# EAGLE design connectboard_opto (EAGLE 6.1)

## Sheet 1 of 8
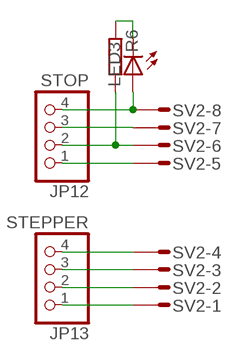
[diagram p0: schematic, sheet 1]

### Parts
JP12  STOP  PINHD-1X04_2.54-S  [1X04-S]
JP13  STEPPER  PINHD-1X04_2.54-S  [1X04-S]
LED3  LED3MM  [LED3MM]
R6  R-EU0207/10  [0207/10]
SV2  ML10E  [ML10]

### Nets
MYZ-1: JP13.1 SV2.1
MYZ-2: JP13.2 SV2.2
MYZ-3: JP13.3 SV2.3
MYZ-4: JP13.4 SV2.4
N$5: LED3.K(C) R6.1
YZ-LEDA: JP12.4 LED3.A SV2.8
YZ-LEDC: JP12.3 SV2.7
YZ-SW: JP12.2 R6.2 SV2.6
YZ-SW-GND: JP12.1 SV2.5
Unconnected: SV2.9 SV2.10

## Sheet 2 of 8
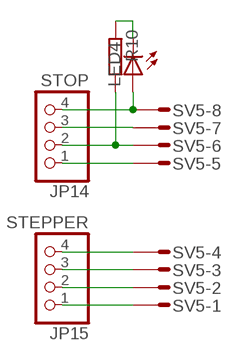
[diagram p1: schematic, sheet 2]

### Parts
JP14  STOP  PINHD-1X04_2.54-S  [1X04-S]
JP15  STEPPER  PINHD-1X04_2.54-S  [1X04-S]
LED4  LED3MM  [LED3MM]
R10  R-EU0207/10  [0207/10]
SV5  ML10E  [ML10]

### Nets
MYZ-5: JP15.1 SV5.1
MYZ-6: JP15.2 SV5.2
MYZ-7: JP15.3 SV5.3
MYZ-8: JP15.4 SV5.4
N$6: LED4.K(C) R10.1
YZ-LEDA1: JP14.4 LED4.A SV5.8
YZ-LEDC1: JP14.3 SV5.7
YZ-SW1: JP14.2 R10.2 SV5.6
YZ-SW-GND1: JP14.1 SV5.5
Unconnected: SV5.9 SV5.10

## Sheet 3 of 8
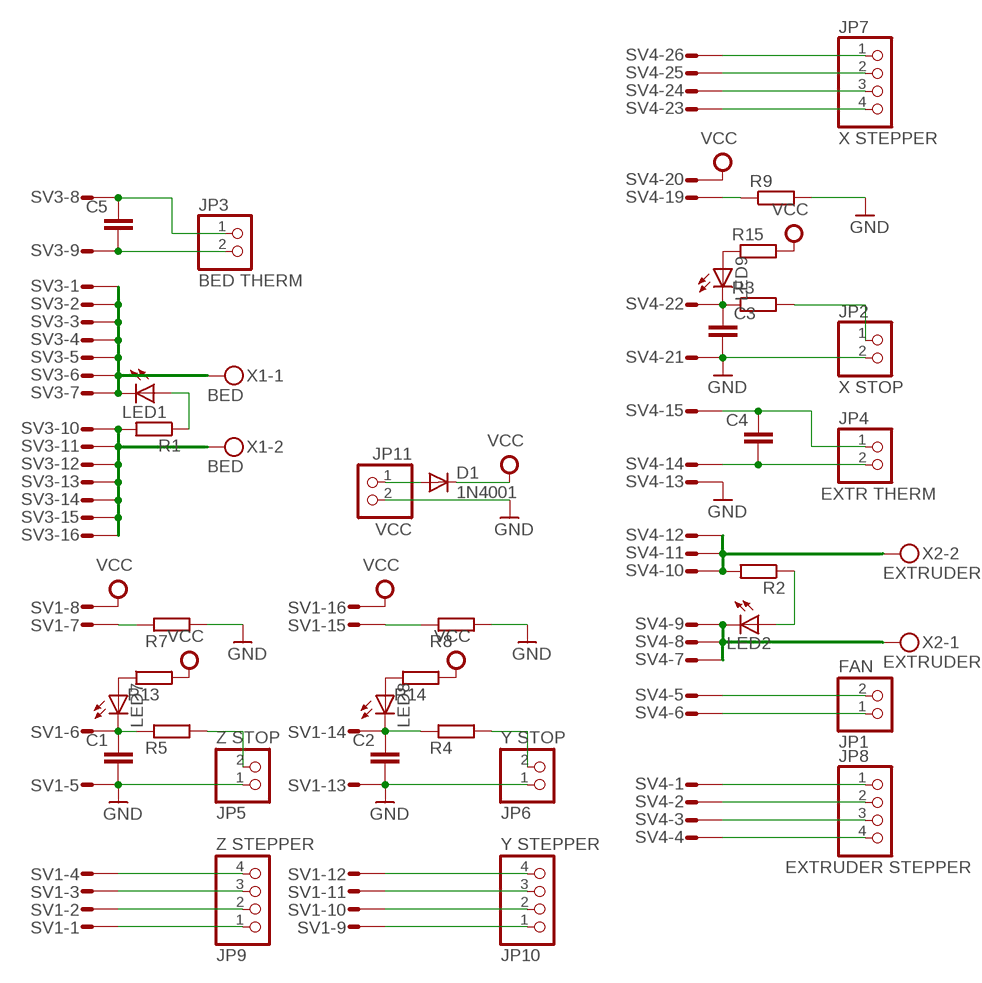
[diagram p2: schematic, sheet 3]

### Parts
C1  C-EU025-024X044  [C025-024X044]
C2  C-EU025-024X044  [C025-024X044]
C3  C-EU025-024X044  [C025-024X044]
C4  C-EU025-024X044  [C025-024X044]
C5  C-EU025-024X044  [C025-024X044]
D1  1N4001  [DO41-10]
JP1  FAN  PINHD-1X02_2.54-S  [1X02-S]
JP2  X STOP  PINHD-1X02_2.54  [1X02]
JP3  BED THERM  PINHD-1X02_2.54  [1X02]
JP4  EXTR THERM  PINHD-1X02_2.54  [1X02]
JP5  Z STOP  PINHD-1X02_2.54-S  [1X02-S]
JP6  Y STOP  PINHD-1X02_2.54-S  [1X02-S]
JP7  X STEPPER  PINHD-1X04_2.54-S  [1X04-S]
JP8  EXTRUDER STEPPER  PINHD-1X04_2.54-S  [1X04-S]
JP9  Z STEPPER  PINHD-1X04_2.54-S  [1X04-S]
JP10  Y STEPPER  PINHD-1X04_2.54-S  [1X04-S]
JP11  VCC  PINHD-1X02_2.54-S  [1X02-S]
LED1  LED3MM  [LED3MM]
LED2  LED3MM  [LED3MM]
LED7  LED3MM  [LED3MM]
LED8  LED3MM  [LED3MM]
LED9  LED3MM  [LED3MM]
R1  R-EU0207/10  [0207/10]
R2  R-EU0207/10  [0207/10]
R3  R-EU0207/2V  [0207/2V]
R4  R-EU0207/2V  [0207/2V]
R5  R-EU0207/2V  [0207/2V]
R7  R-EU0207/2V  [0207/2V]
R8  R-EU0207/2V  [0207/2V]
R9  R-EU0207/2V  [0207/2V]
R13  R-EU0207/2V  [0207/2V]
R14  R-EU0207/2V  [0207/2V]
R15  R-EU0207/10  [0207/10]
SV1  ML16E  [ML16]
SV3  ML16E  [ML16]
SV4  ML26E  [ML26]
X1  BED  MKDSN1,5/2-5,08  [MKDSN1,5/2-5,08]
X2  EXTRUDER  MKDSN1,5/2-5,08  [MKDSN1,5/2-5,08]

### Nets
GND: C1.2 C2.2 C3.2 JP2.2 JP5.1 JP6.1 JP11.2 R7.2 R8.2 R9.2 SV1.5 SV1.13 SV4.13 SV4.21
MEXT-1: JP8.1 SV4.1
MEXT-2: JP8.2 SV4.2
MEXT-3: JP8.3 SV4.3
MEXT-4: JP8.4 SV4.4
MX-1: JP7.1 SV4.26
MX-2: JP7.2 SV4.25
MX-3: JP7.3 SV4.24
MX-4: JP7.4 SV4.23
MY-1: JP10.1 SV1.9
MY-2: JP10.2 SV1.10
MY-3: JP10.3 SV1.11
MY-4: JP10.4 SV1.12
MZ-1: JP9.1 SV1.1
MZ-2: JP9.2 SV1.2
MZ-3: JP9.3 SV1.3
MZ-4: JP9.4 SV1.4
N$1: C5.2 JP3.2 SV3.9
N$2: C5.1 JP3.1 SV3.8
N$3: LED1.K(C) SV3.1 SV3.2 SV3.3 SV3.4 SV3.5 SV3.6 SV3.7 X1.1
N$4: R1.2 SV3.10 SV3.11 SV3.12 SV3.13 SV3.14 SV3.15 SV3.16 X1.2
N$9: JP5.2 R5.2
N$11: JP6.2 R4.2
N$21: C4.2 JP4.2 SV4.14
N$22: C4.1 JP4.1 SV4.15
N$23: JP1.1 SV4.6
N$24: JP1.2 SV4.5
N$25: R2.2 SV4.10 SV4.11 SV4.12 X2.2
N$26: LED7.A R13.1
N$27: LED8.A R14.1
N$28: D1.A JP11.1
N$29: LED9.A R15.1
N$30: JP2.1 R3.2
N$32: LED2.K(C) SV4.7 SV4.8 SV4.9 X2.1
N$33: LED1.A R1.1
N$34: LED2.A R2.1
VCC: D1.C R13.2 R14.2 R15.2 SV1.8 SV1.16 SV4.20
X-LEDC: R9.1 SV4.19
X-SW: C3.1 LED9.K(C) R3.1 SV4.22
Y-LEDC: R8.1 SV1.15
Y-SW: C2.1 LED8.K(C) R4.1 SV1.14
Z-LEDC: R7.1 SV1.7
Z-SW: C1.1 LED7.K(C) R5.1 SV1.6
Unconnected: SV4.16 SV4.17 SV4.18

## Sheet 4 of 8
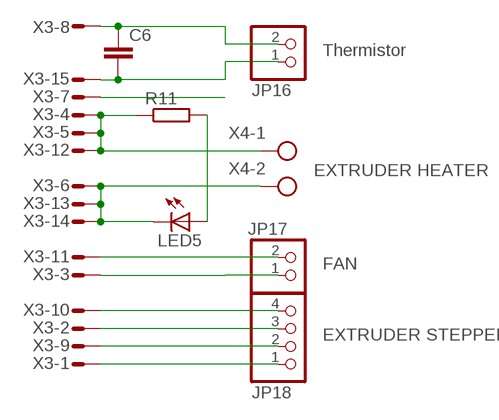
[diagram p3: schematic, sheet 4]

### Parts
C6  C-EU025-024X044  [C025-024X044]
JP16  Thermistor  PINHD-1X02_2.54-90°-S  [1X02/90-S]
JP17  FAN  PINHD-1X02_2.54-90°-S  [1X02/90-S]
JP18  EXTRUDER STEPPER  PINHD-1X04_2.54-90°-S  [1X04/90-S]
LED5  LED3MM  [LED3MM]
R11  R-EU0207/10  [0207/10]
X3  M15HS  [M15H]
X4  EXTRUDER HEATER  MKDSN1,5/2-5,08  [MKDSN1,5/2-5,08]

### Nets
N$7: JP18.1 X3.1
N$8: JP18.3 X3.2
N$10: JP18.2 X3.9
N$12: JP18.4 X3.10
N$13: JP17.1 X3.3
N$14: JP17.2 X3.11
N$15: C6.2 JP16.1 X3.15
N$16: C6.1 JP16.2 X3.8
N$17: R11.1 X3.4 X3.5 X3.12 X4.1
N$18: LED5.K(C) X3.6 X3.13 X3.14 X4.2
N$19: LED5.A R11.2
SHIELD: X3.7

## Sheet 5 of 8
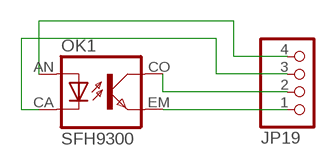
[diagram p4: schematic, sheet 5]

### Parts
JP19  PINHD-1X04_2.54-90°L-S  [1X04/90L-S]
OK1  SFH9300  [SFH9300]

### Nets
LEDA: JP19.4 OK1.AN(A)
LEDC: JP19.3 OK1.CA(C)
SW: JP19.2 OK1.CO(COL)
SW-GND: JP19.1 OK1.EM(EMIT)

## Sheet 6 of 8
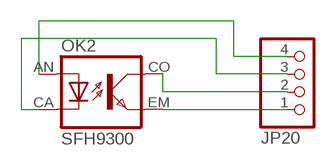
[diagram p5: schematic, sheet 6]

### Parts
JP20  PINHD-1X04_2.54-90°L-S  [1X04/90L-S]
OK2  SFH9300  [SFH9300]

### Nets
LEDA1: JP20.4 OK2.AN(A)
LEDC1: JP20.3 OK2.CA(C)
SW1: JP20.2 OK2.CO(COL)
SW-GND1: JP20.1 OK2.EM(EMIT)

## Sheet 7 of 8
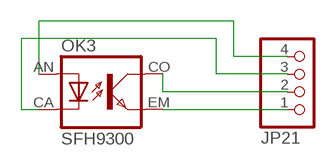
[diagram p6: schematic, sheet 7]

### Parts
JP21  PINHD-1X04_2.54-90°L-S  [1X04/90L-S]
OK3  SFH9300  [SFH9300]

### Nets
LEDA2: JP21.4 OK3.AN(A)
LEDC2: JP21.3 OK3.CA(C)
SW2: JP21.2 OK3.CO(COL)
SW-GND2: JP21.1 OK3.EM(EMIT)

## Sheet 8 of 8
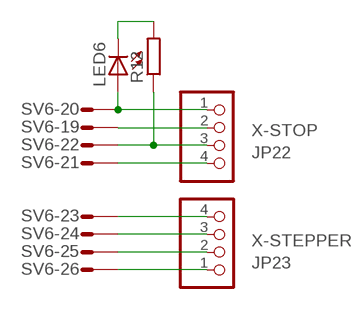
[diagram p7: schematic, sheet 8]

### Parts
JP22  X-STOP  PINHD-1X04_2.54-90°L-S  [1X04/90L-S]
JP23  X-STEPPER  PINHD-1X04_2.54-90°-S  [1X04/90-S]
LED6  LED3MM  [LED3MM]
R12  R-EU0207/10  [0207/10]
SV6  ML26LE  [ML26L]

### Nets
N$20: LED6.K(C) R12.2
X-LEDA: JP22.1 LED6.A SV6.20
X-LEDC1: JP22.2 SV6.19
X-SW1: JP22.3 R12.1 SV6.22
X-SW-GND: JP22.4 SV6.21
XM1: JP23.1 SV6.26
XM2: JP23.2 SV6.25
XM3: JP23.3 SV6.24
XM4: JP23.4 SV6.23
Unconnected: SV6.1 SV6.2 SV6.3 SV6.4 SV6.5 SV6.6 SV6.7 SV6.8 SV6.9 SV6.10 SV6.11 SV6.12 SV6.13 SV6.14 SV6.15 SV6.16 SV6.17 SV6.18

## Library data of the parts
C1-C6 = rcl-2:C-EU: CAPACITOR, European symbol
D1 = diode:1N400*: DIODE
JP1-JP6 JP11 JP16 JP17 = con-pinhead-2:PINHD-1X02: PIN HEADER
JP7-JP10 JP12-JP15 JP18-JP23 = con-pinhead-2:PINHD-1X04: PIN HEADER
LED1-LED9 = led:LED: LED
OK1-OK3 = opto-siemens:SFH9*: Slotted Interrupter / Gabellichtschranke Source: http://www.osram.convergy.de/
R1-R15 = rcl-2:R-EU: RESISTOR, European symbol
SV1 SV3 = con-dil:ML16?E: HARTING
SV2 SV5 = con-dil:ML10?E: HARTING
SV4 SV6 = con-dil:ML26?E: HARTING
X1 X2 X4 = con-phoenix-508:MKDSN1,5/2-5,08: MKDSN 1,5/ 2-5,08 Printklemme
X3 = con-subd:M15?S: SUB-D

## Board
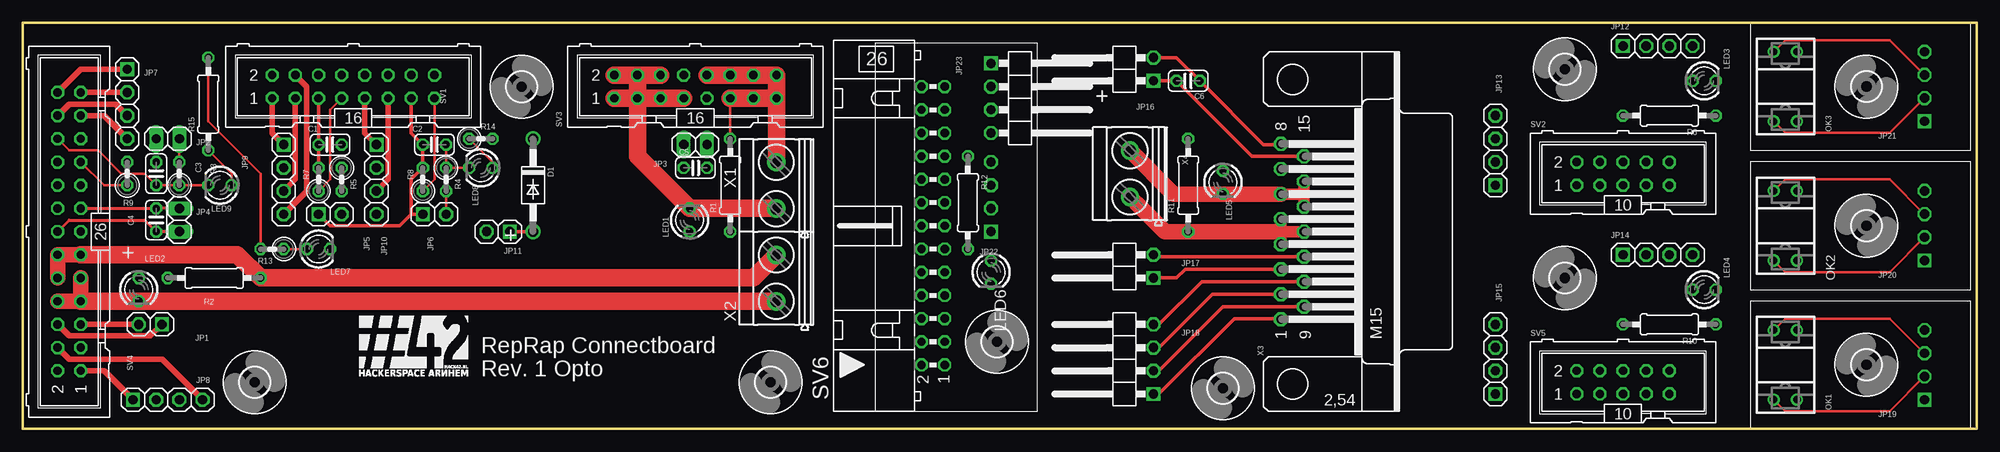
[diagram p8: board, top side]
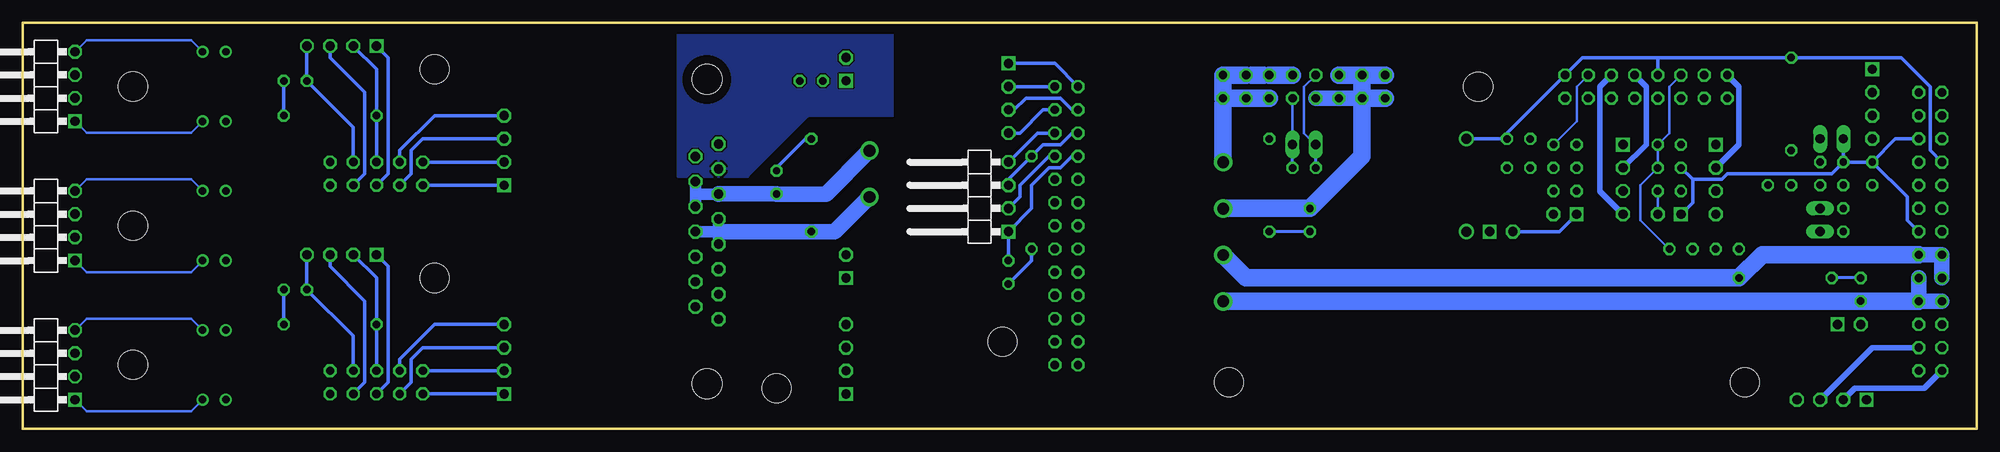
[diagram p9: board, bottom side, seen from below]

Size 214 x 44.45 mm. Coordinates in mm from the lower left corner, seen from the top.
Outline: 0,0 214,0 214,44.45 0,44.45 0,0
Copper layers (1*16): Top 0.035mm / dielectric 1.5mm / Bottom 0.035mm
Design rules: minimum track width 10mil, minimum drill 24mil, track to track 8mil, track to pad 8mil, pad to pad 8mil, via to via 8mil, smd to smd 8mil, copper to edge 40mil, drill to drill 8mil, minimum pad ring 10mil, minimum via ring 8mil, stop-mask expansion 4mil, vias tented up to drill 0mil, thermal gap 10mil

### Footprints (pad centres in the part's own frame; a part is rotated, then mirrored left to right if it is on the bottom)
C025-024X044 = drill 0.813 octagon: 1 -1.27,0; 2 1.27,0
DO41-10 = drill 1.118: A 5.08,0; C -5.08,0
1X02-S = drill 1.016 square: 1 -1.27,0 | drill 1.016 octagon: 2 1.27,0
1X02 = drill 1.016 long: 1 -1.27,0; 2 1.27,0
1X04-S = drill 1.016 square: 1 -3.81,0 | drill 1.016 octagon: 2 -1.27,0; 3 1.27,0; 4 3.81,0
1X02/90-S = drill 1.016 square: 1 -2.54,-3.81 | drill 1.016 octagon: 2 0,-3.81
1X04/90-S = drill 1.016 square: 1 -3.81,-3.81 | drill 1.016 octagon: 2 -1.27,-3.81; 3 1.27,-3.81; 4 3.81,-3.81
1X04/90L-S = drill 1.016 square: 1 3.81,-3.81 | drill 1.016 octagon: 2 1.27,-3.81; 3 -1.27,-3.81; 4 -3.81,-3.81
LED3MM = drill 0.813 octagon: A -1.27,0; K 1.27,0
SFH9300 = drill 0.813: AN -3.81,1.27; CA -3.81,-1.27; CO 3.81,-1.27; EM 3.81,1.27
0207/10 = drill 0.813 octagon: 1 -5.08,0; 2 5.08,0
0207/2V = drill 0.813 octagon: 1 -1.27,0; 2 1.27,0
ML16 = drill 0.914 octagon: 1 -8.89,-1.27; 2 -8.89,1.27; 3 -6.35,-1.27; 4 -6.35,1.27; 5 -3.81,-1.27; 6 -3.81,1.27; 7 -1.27,-1.27; 8 -1.27,1.27; 9 1.27,-1.27; 10 1.27,1.27; 11 3.81,-1.27; 12 3.81,1.27; 13 6.35,-1.27; 14 6.35,1.27; 15 8.89,-1.27; 16 8.89,1.27
ML10 = drill 0.914 octagon: 1 -5.08,-1.27; 2 -5.08,1.27; 3 -2.54,-1.27; 4 -2.54,1.27; 5 0,-1.27; 6 0,1.27; 7 2.54,-1.27; 8 2.54,1.27; 9 5.08,-1.27; 10 5.08,1.27
ML26 = drill 0.914 octagon: 1 -15.24,-1.27; 2 -15.24,1.27; 3 -12.7,-1.27; 4 -12.7,1.27; 5 -10.16,-1.27; 6 -10.16,1.27; 7 -7.62,-1.27; 8 -7.62,1.27; 9 -5.08,-1.27; 10 -5.08,1.27; 11 -2.54,-1.27; 12 -2.54,1.27; 13 0,-1.27; 14 0,1.27; 15 2.54,-1.27; 16 2.54,1.27; 17 5.08,-1.27; 18 5.08,1.27; 19 7.62,-1.27; 20 7.62,1.27; 21 10.16,-1.27; 22 10.16,1.27; 23 12.7,-1.27; 24 12.7,1.27; 25 15.24,-1.27; 26 15.24,1.27
ML26L = drill 0.914 octagon: 1 -15.24,-1.27; 2 -15.24,1.27; 3 -12.7,-1.27; 4 -12.7,1.27; 5 -10.16,-1.27; 6 -10.16,1.27; 7 -7.62,-1.27; 8 -7.62,1.27; 9 -5.08,-1.27; 10 -5.08,1.27; 11 -2.54,-1.27; 12 -2.54,1.27; 13 0,-1.27; 14 0,1.27; 15 2.54,-1.27; 16 2.54,1.27; 17 5.08,-1.27; 18 5.08,1.27; 19 7.62,-1.27; 20 7.62,1.27; 21 10.16,-1.27; 22 10.16,1.27; 23 12.7,-1.27; 24 12.7,1.27; 25 15.24,-1.27; 26 15.24,1.27
3,2 = hole 3.2: 0,0
MKDSN1,5/2-5,08 = drill 1.3 pad 2: 1 -2.561,0.025; 2 2.519,0.025
M15H = drill 1.016 octagon: 1 -9.601,1.27; 2 -6.858,1.27; 3 -4.115,1.27; 4 -1.372,1.27; 5 1.372,1.27; 6 4.115,1.27; 7 6.858,1.27; 8 9.601,1.27; 9 -8.23,-1.27; 10 -5.486,-1.27; 11 -2.743,-1.27; 12 0,-1.27; 13 2.743,-1.27; 14 5.486,-1.27; 15 8.23,-1.27 | hole 3.302: 16.662,0; -16.662,0

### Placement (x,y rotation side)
C1  33.66,31.11 180 top
C2  45.09,31.11 180 top
C3  14.61,27.94 90 top
C4  14.61,22.86 270 top
C5  73.66,28.57 0 top
C6  127.64,38.1 180 top
D1  55.88,26.67 270 top
JP1  13.97,11.43 180 top
JP2  15.88,31.75 180 top
JP3  73.66,31.11 0 top
JP4  17.14,22.86 270 top
JP5  33.66,23.5 0 top
JP6  45.09,23.5 0 top
JP7  11.43,35.56 270 top
JP8  15.88,3.17 0 top
JP9  28.57,27.3 270 top
JP10  38.73,27.3 270 top
JP11  52.07,21.59 180 top
JP12  179.07,41.91 0 top
JP13  161.29,30.48 90 top
JP14  179.07,19.05 0 top
JP15  161.29,7.62 90 top
JP16  120.02,40.64 90 top
JP17  120.02,19.05 90 top
JP18  120.02,7.62 90 top
JP19  212.09,7 270 top
JP20  212.09,22.23 270 top
JP21  212.09,37.48 270 top
JP22  109.86,25.4 270 top
JP23  109.86,36.2 270 top
LED1  73.03,22.86 90 top
LED2  12.7,15.24 270 top
LED3  184.15,38.1 0 top
LED4  184.15,15.24 0 top
LED5  131.44,26.99 270 top
LED6  106.05,17.14 270 top
LED7  32.38,19.68 0 top
LED8  50.16,28.57 180 top
LED9  21.59,26.67 180 top
OK1  193.04,7 270 top
OK2  193.04,22.23 270 top
OK3  193.04,37.48 270 top
R1  77.47,26.67 90 top
R2  20.95,16.51 0 top
R3  17.14,27.94 90 top
R4  46.35,27.3 270 top
R5  34.92,27.3 270 top
R6  180.34,34.29 180 top
R7  32.38,27.3 90 top
R8  43.81,27.3 90 top
R9  11.43,27.94 90 top
R10  180.34,11.43 180 top
R11  127.64,26.67 90 top
R12  103.5,24.77 270 top
R13  27.3,19.68 180 top
R14  50.16,31.75 0 top
R15  20.32,35.56 90 top
SV1  36.2,37.47 0 top
SV2  175.26,27.94 0 top
SV3  73.66,37.47 0 top
SV4  5.08,21.59 90 top
SV5  175.26,5.08 0 top
SV6  99.69,22.23 90 top
U$1  [3,2]  25.4,5.08 0 top
U$2  [3,2]  81.92,5.08 0 top
U$3  [3,2]  168.91,39.37 90 top
U$4  [3,2]  54.61,37.47 0 top
U$5  [3,2]  168.91,16.51 90 top
U$6  [3,2]  131.44,4.45 0 top
U$7  [3,2]  201.93,7 90 top
U$8  [3,2]  201.93,22.23 90 top
U$9  [3,2]  201.93,37.48 90 top
U$10  [3,2]  106.68,9.53 0 top
U$11  [LOGO_HACK42-12X7]  36.83,5.71 0 top
X1  82.55,26.67 90 top
X2  82.55,16.51 90 top
X3  139.06,21.59 90 top
X4  121.28,27.94 90 top

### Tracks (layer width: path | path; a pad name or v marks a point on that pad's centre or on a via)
GND
  Top 0.406: SV1.13 42.55,32.38 C2.2 R8.2 42.55,27.3 42.55,23.5 | R7.2 C1.2 SV1.5 | JP5.1 33.66,22.23 41.27,22.23 42.55,23.5 | JP6.1 42.55,23.5
  Bottom 0.406: C3.2 R9.2 | SV4.21 8.89,31.75 R9.2 | C3.2 JP2.2 | 31.11,27.3 R7.2 | 31.11,27.3 31.11,24.77 JP5.1 | C3.2 15.88,27.94 27.3,27.94 27.94,27.3 31.11,27.3 | JP11.2 45.72,21.59 JP6.1 | R9.2 7.62,25.4 7.62,22.86 SV4.13
LEDA
  Bottom 0.254: OK1.AN 195.58,12.07 207.01,12.07 JP19.4
LEDA1
  Bottom 0.254: OK2.AN 195.58,27.32 207.01,27.32 JP20.4
LEDA2
  Bottom 0.254: OK3.AN 195.58,42.55 207.01,42.55 JP21.4
LEDC
  Top 0.254: OK1.CA 193.04,12.07 204.47,12.07 JP19.3
LEDC1
  Top 0.254: OK2.CA 193.04,27.32 204.47,27.32 JP20.3
LEDC2
  Top 0.254: OK3.CA 193.04,42.55 204.47,42.55 JP21.3
MEXT-1
  Top 0.61: SV4.1 8.89,6.35 JP8.1
MEXT-2
  Bottom 0.61: SV4.2 5.71,4.45 13.34,4.45 JP8.2
MEXT-3
  Bottom 0.61: SV4.3 11.43,8.89 JP8.3
MEXT-4
  Top 0.61: SV4.4 5.08,7.62 15.24,7.62 JP8.4
MX-1
  Top 0.61: SV4.26 6.35,39.37 JP7.1
MX-2
  Top 0.61: JP7.2 SV4.25
MX-3
  Top 0.61: SV4.24 5.08,35.56 10.16,35.56 JP7.3
MX-4
  Top 0.61: SV4.23 8.89,34.29 JP7.4
MY-1
  Top 0.61: SV1.9 37.47,32.38 JP10.1
MY-2
  Bottom 0.61: SV1.10 36.2,37.47 36.2,31.11 JP10.2
MY-3
  Top 0.61: SV1.11 40.01,27.3 JP10.3
MY-4
  Bottom 0.61: SV1.12 41.27,37.47 41.27,26.04 JP10.4
MYZ-1
  Bottom 0.406: SV2.1 JP13.1
MYZ-2
  Bottom 0.406: JP13.2 SV2.2
MYZ-3
  Bottom 0.406: JP13.3 170.18,31.75 171.45,30.48 171.45,27.94 SV2.3
MYZ-4
  Bottom 0.406: JP13.4 168.91,34.29 172.72,30.48 SV2.4
MYZ-5
  Bottom 0.406: SV5.1 JP15.1
MYZ-6
  Bottom 0.406: JP15.2 SV5.2
MYZ-7
  Bottom 0.406: JP15.3 170.18,8.89 171.45,7.62 171.45,5.08 SV5.3
MYZ-8
  Bottom 0.406: JP15.4 168.91,11.43 172.72,7.62 SV5.4
MZ-1
  Top 0.61: SV1.1 27.3,32.38 JP9.1
MZ-2
  Bottom 0.61: SV1.2 26.04,37.47 26.04,31.11 JP9.2
MZ-3
  Top 0.61: SV1.3 29.84,27.3 JP9.3
MZ-4
  Top 0.61: SV1.4 31.11,37.47 31.11,26.04 JP9.4
N$1
  Bottom 0.254: JP3.2 SV3.9
  Bottom 0.305: C5.2 JP3.2
N$2
  Bottom 0.254: SV3.8 73.66,37.47 73.66,32.38 JP3.1
  Bottom 0.305: C5.1 JP3.1
N$3
  Top 1.93: SV3.2 SV3.4 | SV3.4 SV3.6 | SV3.1 SV3.3 | SV3.3 SV3.7 | SV3.4 SV3.3 | SV3.3 67.31,29.84 LED1.K 82.55,24.13
  Bottom 1.27: 66.67,36.2 SV3.3 SV3.5 SV3.7 | 82.55,24.13 X1.1
  Bottom 1.676: SV3.7 SV3.3
  Bottom 1.93: SV3.4 SV3.6 | SV3.1 SV3.3 | SV3.4 SV3.3 | SV3.4 SV3.2 | SV3.3 67.31,29.84 LED1.K 82.55,24.13
N$4
  Top 0.254: SV3.11 R1.2
  Top 1.93: 82.55,29.21 SV3.15 | SV3.15 SV3.16 SV3.14 SV3.12 SV3.10 | SV3.11 SV3.13 SV3.15
  Bottom 0.406: 82.55,29.21 82.53,29.21 X1.2
  Bottom 1.27: 79.38,38.73 SV3.14 | SV3.12 78.11,38.73 | 82.55,35.56 SV3.15 | 82.55,29.21 X1.2
  Bottom 1.93: SV3.11 SV3.13 SV3.15 SV3.16 SV3.14 | SV3.10 SV3.12 | 78.11,38.73 79.38,38.73 | 82.55,29.21 82.55,35.56
N$5
  Bottom 0.406: R6.1 LED3.K
N$6
  Bottom 0.406: R10.1 LED4.K
N$7
  Top 0.406: JP18.1 124.46,3.81 132.72,12.06 137.79,12.06 X3.1
N$8
  Top 0.406: JP18.3 124.46,8.89 130.3,14.73 X3.2 137.92,14.73
N$9
  Bottom 0.254: JP5.2 R5.2
N$10
  Top 0.254: 140.34,13.34 X3.9
  Top 0.406: JP18.2 124.46,6.35 131.44,13.34 140.34,13.34
N$11
  Top 0.254: JP6.2 R4.2
N$12
  Top 0.406: JP18.4 124.46,11.43 129.13,16.1 X3.10
N$13
  Top 0.406: X3.3 127.33,17.48 126.36,16.51 JP17.1
N$14
  Top 0.406: JP17.2 124.26,18.85 X3.11
N$15
  Top 0.254: 140.34,29.84 X3.15
  Top 0.406: JP16.1 C6.2 134.62,29.84 140.34,29.84
N$16
  Top 0.254: 137.79,31.11 X3.8
  Top 0.406: JP16.2 126.36,40.64 C6.1 135.89,31.11 137.79,31.11
N$17
  Top 0.254: 137.79,20.32 X3.4
  Top 0.813: 137.79,22.86 X3.5
  Top 1.27: 137.79,21.59 137.79,20.32 | 137.79,21.59 X3.12 | 137.79,21.59 137.79,22.86
  Top 1.676: X4.1 121.92,24.77 125.09,21.59 R11.1 137.79,21.59
  Bottom 1.27: 137.79,21.59 137.79,22.86 | 137.79,21.59 137.79,20.32 | X3.12 137.79,21.59
  Bottom 1.676: 121.28,25.4 125.09,21.59 137.79,21.59
N$18
  Top 0.254: LED5.K 131.44,25.7
  Top 0.813: 121.28,30.48 X4.2
  Top 1.27: X3.14 140.34,25.7 | X3.13 140.34,25.7 | 140.34,25.7 X3.6
  Top 1.676: 121.28,30.48 126.03,25.7 131.44,25.7 X3.6
  Bottom 0.254: 130.18,25.08 130.18,25.7 | 121.44,30.32 121.28,30.16 X4.2
  Bottom 1.27: 140.34,24.13 140.34,25.7 | X3.6 140.34,25.7 | 140.34,25.7 X3.14
  Bottom 1.676: LED5.K 137.78,25.72 X3.6 | 131.44,25.7 130.18,25.7 126.03,25.7 121.44,30.32 121.28,30.48
N$19
  Bottom 0.406: R11.2 128.27,31.75 131.44,28.57 LED5.A
N$20
  Bottom 0.406: R12.2 103.5,18.41 LED6.K
N$21
  Top 0.305: JP4.2 C4.2 13.34,22.86 5.08,22.86 SV4.14
N$22
  Top 0.305: JP4.1 C4.1 SV4.15
N$23
  Top 0.61: SV4.6 5.08,10.16 13.97,10.16 JP1.1
N$24
  Top 0.61: JP1.2 SV4.5
N$25
  Top 1.676: SV4.10 SV4.12 SV4.11
  Top 1.93: 82.55,19.05 80.01,16.51 R2.2 23.5,19.05 SV4.11
  Bottom 1.676: SV4.11 SV4.12 SV4.10
  Bottom 1.93: SV4.11 23.5,19.05 R2.2 80.01,16.51 81.92,18.41 X2.2
N$26
  Top 0.254: R13.1 LED7.A
N$27
  Top 0.254: R14.1 51.44,29.21 LED8.A
N$28
  Top 0.406: D1.A JP11.1
N$29
  Top 0.254: LED9.A 22.86,27.94 R15.1
N$30
  Top 0.254: JP2.1 R3.2
N$32
  Top 1.676: SV4.9 SV4.7 SV4.8
  Top 1.93: SV4.7 LED2.K 82.55,13.97
  Bottom 1.676: SV4.9 SV4.7 SV4.8
  Bottom 1.93: SV4.7 LED2.K 81.92,13.97 X2.1
N$33
  Bottom 0.305: LED1.A R1.1
N$34
  Bottom 0.305: LED2.A R2.1
SHIELD
  pour Bottom: 118.75,34.29 127.95,34.29 134.62,27.62 142.24,27.62 142.24,43.18 118.75,43.18
SW
  Top 0.254: OK1.CO 193.04,1.92 204.47,1.92 JP19.2
SW1
  Top 0.254: OK2.CO 193.04,17.16 204.47,17.16 JP20.2
SW2
  Top 0.254: OK3.CO 193.04,32.4 204.47,32.4 JP21.2
SW-GND
  Bottom 0.254: OK1.EM 195.58,1.92 207.01,1.92 JP19.1
SW-GND1
  Bottom 0.254: OK2.EM 195.58,17.16 207.01,17.16 JP20.1
SW-GND2
  Bottom 0.254: OK3.EM 195.58,32.4 207.01,32.4 JP21.1
VCC
  Top 0.254: R13.2 26.04,27.94 20.32,33.66 R15.2
  Bottom 0.406: SV4.20 5.08,30.48 5.08,37.47 8.26,40.64 R15.2 34.92,40.64 | SV1.8 34.92,40.64 | 34.92,40.64 43.18,40.64 SV1.16 51.44,32.38 R14.2 D1.C
X-LEDA
  Bottom 0.406: SV6.20 99.06,29.84 100.33,28.57 101.6,28.57 103.5,26.67 103.5,24.13 JP22.1 LED6.A
X-LEDC
  Top 0.254: R9.1 8.89,26.67 SV4.19
X-LEDC1
  Bottom 0.406: JP22.2 104.78,25.4 104.78,26.67 101.6,29.84 SV6.19
X-SW
  Top 0.254: SV4.22 5.08,30.48 8.26,30.48 10.79,27.94 13.34,27.94 C3.1 R3.1 LED9.K
X-SW1
  Bottom 0.406: JP22.3 106.05,27.3 R12.1 102.23,31.11 100.33,31.11 99.06,32.38 SV6.22
X-SW-GND
  Bottom 0.406: JP22.4 102.87,32.38 SV6.21
XM1
  Bottom 0.406: SV6.26 100.97,40.01 JP23.1
XM2
  Bottom 0.406: JP23.2 SV6.25
XM3
  Bottom 0.406: JP23.3 105.41,34.92 104.14,36.2 100.33,36.2 99.06,34.92 SV6.24
XM4
  Bottom 0.406: SV6.23 102.23,34.92 104.78,32.38 JP23.4
Y-LEDC
  Top 0.254: R8.1 45.09,27.3 SV1.15
Y-SW
  Top 0.254: C2.1 R4.1 LED8.K
  Bottom 0.254: SV1.14 43.81,37.47 43.81,33.66 C2.1
YZ-LEDA
  Bottom 0.406: JP12.4 LED3.A 177.8,33.02 SV2.8
YZ-LEDA1
  Bottom 0.406: JP14.4 LED4.A 177.8,10.16 SV5.8
YZ-LEDC
  Bottom 0.406: JP12.3 180.34,40.64 176.53,36.83 176.53,27.94 SV2.7
YZ-LEDC1
  Bottom 0.406: JP14.3 180.34,17.78 176.53,13.97 176.53,5.08 SV5.7
YZ-SW
  Bottom 0.406: JP12.2 175.26,39.37 R6.2 SV2.6
YZ-SW1
  Bottom 0.406: JP14.2 175.26,16.51 R10.2 SV5.6
YZ-SW-GND
  Bottom 0.406: JP12.1 173.99,40.64 173.99,27.94 SV2.5
YZ-SW-GND1
  Bottom 0.406: JP14.1 173.99,17.78 173.99,5.08 SV5.5
Z-LEDC
  Top 0.254: R7.1 33.66,27.3 33.66,34.92 SV1.7
Z-SW
  Bottom 0.254: SV1.6 33.66,37.47 33.66,32.38 C1.1 R5.1 36.83,26.67 36.83,22.86 LED7.K

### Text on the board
tPlace: RepRap Connectboard | Rev. 1 Opto
tNames: + | + | + | + | + | +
